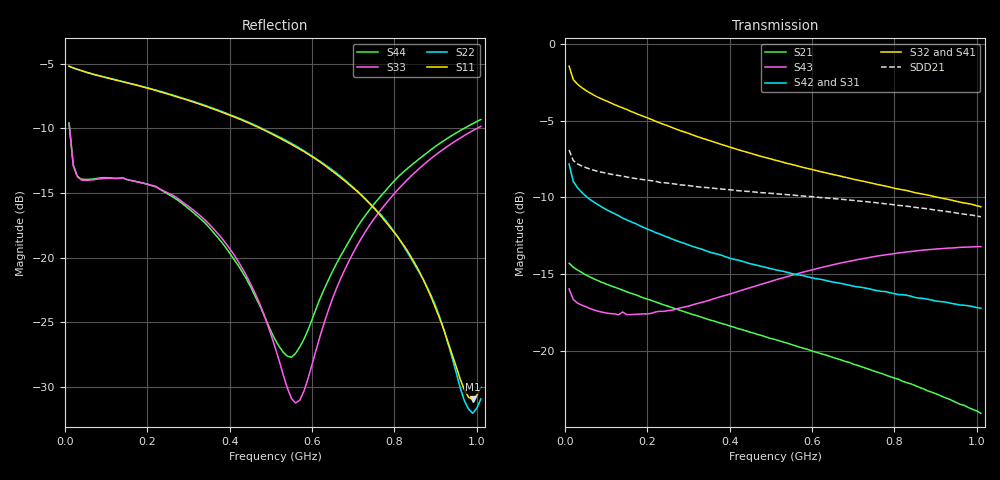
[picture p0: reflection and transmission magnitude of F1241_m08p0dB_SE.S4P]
! Integrated Device Technology
! Corporate Headquarters
! 6024 Silver Creek Valley Road
! San Jose, CA 95138  USA
! Phone:  1-408-284-8200
! Toll Free:  1-800-223-1366
! Webpage:  http://www.idt.com/
! Timing and RF Division
! 515 Groton Road, Suite 102
! Westford, MA 01886-6024
! Device:  F1241
! Description: Dual Intermediate Frequency Digital Variable Gain Amplifier
! Frequency:  10.0 -  500.00 MHz
! Package:  5x5 mm QFN Plastic Package: 32 pin
! Ports:  8 RF, 20 DC
!  Pin  1  = GA3  Pin 17  = RF OUT_B+
!  Pin  2  = GA4  Pin 18  = RF OUT_B-
!  Pin  3  = GA5  Pin 19  = STBY_B
!  Pin  4  = ISET_A  Pin 20  = Ground
!  Pin  5  = ISET_B  Pin 21  = Ground
!  Pin  6  = GB5  Pin 22  = STB_A
!  Pin  7  = GB4  Pin 23  = RF OUT_A-  = Port 4
!  Pin  8  = GB3  Pin 24  = RF OUT_A+  = Port 3
!  Pin  9  = GB2  Pin 25  = NO CONNECT
!  Pin 10  = GB1  Pin 26  = NO CONNECT
!  Pin 11  = RF IN_B+  Pin 27  = VCC
!  Pin 12  = RF IN_B-  Pin 28  = Ground
!  Pin 13  = Ground  Pin 29  = RF IN_A-  = Port 2
!  Pin 14  = VCC  Pin 30  = RF IN_A+  = Port 1
!  Pin 15  = NO CONNECT  Pin 31  = GA1
!  Pin 16  = NO CONNECT  Pin 32  = GA2
! State:  28
! Gain State:  -8.0 dB
! Voltages:  Vcc = +5.00 Volts  Icc approximately 160.0 mA or 80 mA per channel.
! Data:  The device was measured on a custom evaluation board which has
!  individual transmission lines to the RF pins.  Data was collected
!  using a calibrated network analyzer.  The evaluation board was
!  de-embedded using a port reference technique.
!  The reference plane is the edge of the package pin.
!  Only Channel A was measured.
!  This data is in single-ended operation.  If your needs are balanced
!  or differential S-parameters then this file needs to be used a
!  linear simulator.
! Misc:  Lot Code  160028MY
!  Action Tracker AT004
! Date Measured:  2014-08-14
! Date:  2014-08-28  MJV
! Note:
!  Integrated Device Technology supplies this data as a sample of measured
!  data at the package pin for this product.  Your particular data for this
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# Hz S dB R 50
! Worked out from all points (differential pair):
!   101 points, 10 MHz to 1.01 GHz, reference 50 ohm
!   strongest paths, dB at 10 MHz, 260 MHz, 510 MHz, 760 MHz, 1.01 GHz:
!     S32: -1.4, -5.4, -7.6, -9.2, -10.6
!     S41: -1.4, -5.5, -7.7, -9.4, -10.9
!     S42: -7.8, -12.7, -14.7, -16.1, -17.2
!     S31: -7.8, -12.8, -14.8, -16.2, -17.3
!     S43: -16.0, -17.4, -15.4, -13.8, -13.2
!     S21: -14.3, -17.2, -19.3, -21.4, -24.1
!   taken as a pair (ports 2,1 in; 3,4 out), SDD21 dB: -6.9, -9.1, -9.8, -10.4, -11.3
!   lowest |S11| = -31.0 dB at 990 MHz (marker M1), VSWR 1.06, Z = 51.7 + j2.35 ohm
!   |S11| at or under -10 dB: 474 MHz to end of sweep
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1e7  -5.21 -4.4  -14.28 -8.8  -33.30 -2.5  -26.37 5.5
     -14.30 -8.8  -5.20 -4.4  -26.39 5.2  -33.31 -2.6
     -7.85 157.2  -1.45 165.6  -9.65 -44.5  -16.02 177.5
     -1.41 165.7  -7.84 157.3  -15.97 177.5  -9.60 -44.2
4e7  -5.55 -5.9  -14.88 -10.6  -34.09 -8.1  -26.71 -5.0
     -14.89 -10.6  -5.55 -5.7  -26.73 -4.8  -34.09 -8.2
     -9.67 156.6  -2.83 164.8  -14.01 -14.1  -17.08 167.5
     -2.79 164.6  -9.66 156.6  -17.02 167.5  -13.95 -13.6
3.8e8  -8.75 -18.0  -18.19 -36.1  -36.71 -8.7  -28.43 -19.2
       -18.22 -36.2  -8.70 -16.7  -28.27 -18.8  -36.70 -10.4
       -13.90 81.1  -6.55 120.6  -18.47 -10.9  -16.55 108.1
       -6.62 119.3  -13.78 80.3  -16.46 107.9  -18.79 -5.8
5.6e8  -11.44 -21.1  -19.65 -44.4  -36.33 -5.4  -28.50 -24.3
       -19.68 -44.6  -11.36 -19.5  -28.13 -24.8  -36.32 -7.8
       -15.13 51.8  -7.92 103.6  -31.24 55.3  -15.13 83.1
       -8.06 102.1  -15.03 50.3  -15.02 82.8  -27.41 68.4
7.3e8  -15.50 -21.7  -21.06 -51.3  -35.46 -5.5  -28.55 -31.0
       -21.13 -51.4  -15.47 -20.5  -27.91 -32.1  -35.54 -8.8
       -16.05 28.5  -8.98 88.6  -17.97 126.0  -14.10 61.2
       -9.21 87.2  -15.92 26.0  -13.97 61.0  -16.72 120.0
9.9e8  -30.97 53.4  -23.74 -59.0  -33.94 -11.6  -28.73 -42.3
       -23.82 -59.1  -32.04 51.2  -27.80 -44.5  -33.99 -14.0
       -17.21 -0.4  -10.47 66.9  -10.20 122.5  -13.38 32.4
       -10.79 66.1  -17.12 -4.5  -13.23 32.3  -9.65 118.8
1.01e9  -30.02 77.2  -23.97 -59.5  -33.86 -12.4  -28.75 -43.2
        -24.08 -59.3  -30.93 77.9  -27.82 -45.5  -33.87 -15.1
        -17.29 -2.4  -10.61 65.4  -9.85 122.0  -13.36 30.4
        -10.91 64.6  -17.23 -6.2  -13.22 30.3  -9.32 118.3
